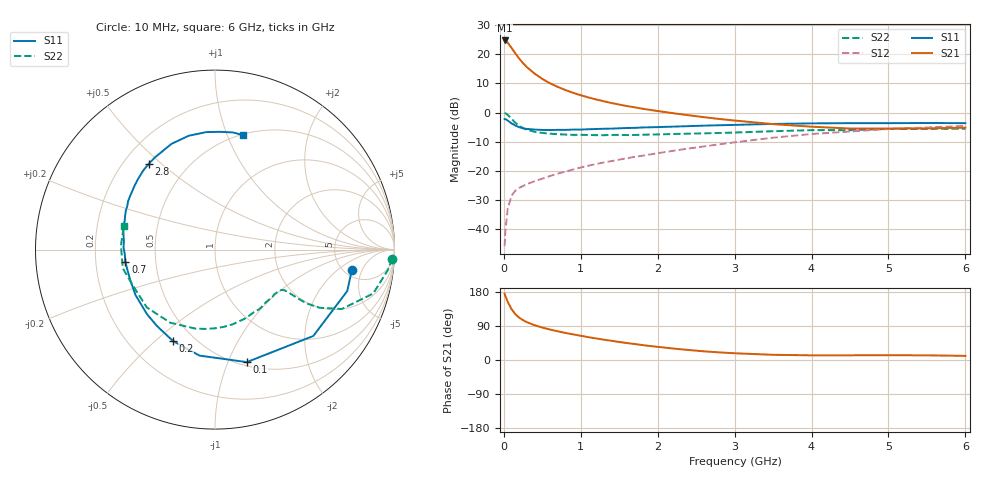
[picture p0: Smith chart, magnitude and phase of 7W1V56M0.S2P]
! Infineon Technologies  Discrete & RF Semiconductors
! BFS17W
! Si NPN RF Bipolar Junction Transistor in SOT323
! VCE = 1.5 V  IC = 6 mA
! Common Emitter S-Parameters:  August  1999
# GHz  S  MA  R  50
!  f  S11  S21  S12  S22
! GHz  MAG  ANG  MAG  ANG  MAG  ANG  MAG  ANG
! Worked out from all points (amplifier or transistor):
!   36 points, 10 MHz to 6 GHz, reference 50 ohm
!   highest |S21| = 24.7 dB at 10 MHz (marker M1)
!   |S21| within 3 dB of that: start of sweep to 111.7 MHz
!   unconditionally stable (mu >= 1): 473.5 MHz to end of sweep
!   at 250 MHz: K = 0.67, MSG = 21.1 dB, |S12| = -25.2 dB
!   at 1.4 GHz: K = 1.29, MAG = 6.7 dB, |S12| = -16.7 dB
!   at 6 GHz: K = 1.11, MAG = -2.3 dB, |S12| = -4.6 dB
!   S11 on the Smith chart (normalised r, x): 10 MHz: 5.81, -3.30; 100 MHz: 0.54, -1.17; 200 MHz: 0.38, -0.57; 700 MHz: 0.33, -0.06; 2.8 GHz: 0.30, +0.46; 6 GHz: 0.51, +1.14
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0.01  0.7708 -8.6  17.2 175.0  0.0051 84.5  0.9887 -2.9
0.02  0.7721 -17.4  17.06 169.0  0.0093 81.9  0.9702 -6.7
0.05  0.7291 -41.3  15.78 153.6  0.0221 70.8  0.9148 -15.5
0.1  0.6514 -74.2  12.83 134.2  0.0373 58.1  0.7802 -25.1
0.15  0.5969 -98.3  10.28 120.7  0.0459 50.5  0.6662 -29.1
0.2  0.5605 -114.7  8.4 111.7  0.051 47.9  0.5913 -30.4
0.25  0.5345 -127.2  7.015 105.1  0.0549 46.3  0.5401 -30.5
0.3  0.5225 -136.5  6.003 99.8  0.0593 46.6  0.5077 -30.4
0.4  0.5101 -150.2  4.638 91.7  0.0663 48.0  0.4661 -30.2
0.5  0.5021 -159.6  3.771 85.6  0.0735 50.4  0.4465 -30.4
0.6  0.5007 -166.6  3.168 80.4  0.0814 52.2  0.4331 -31.3
0.7  0.5039 -172.3  2.752 75.8  0.0894 54.1  0.4245 -32.9
0.9  0.5099 178.5  2.175 67.6  0.1053 56.5  0.4135 -37.0
1.1  0.5165 170.8  1.81 60.2  0.1223 57.8  0.4113 -42.1
1.3  0.5262 164.4  1.558 53.6  0.1391 59.0  0.4082 -47.8
1.6  0.5426 156.2  1.29 44.7  0.164 59.8  0.41 -56.9
2.2  0.5726 141.5  0.973 30.3  0.2205 60.4  0.4279 -76.8
2.8  0.6042 127.5  0.775 20.1  0.284 58.4  0.4457 -97.5
3.5  0.6371 112.4  0.632 13.7  0.3698 53.0  0.4775 -121.5
4.5  0.6566 94.3  0.531 12.4  0.4719 41.1  0.498 -155.3
5.5  0.6604 81.3  0.534 12.3  0.5551 29.5  0.5247 177.5
6  0.6568 76.4  0.55 10.9  0.5884 23.9  0.525 165.5
